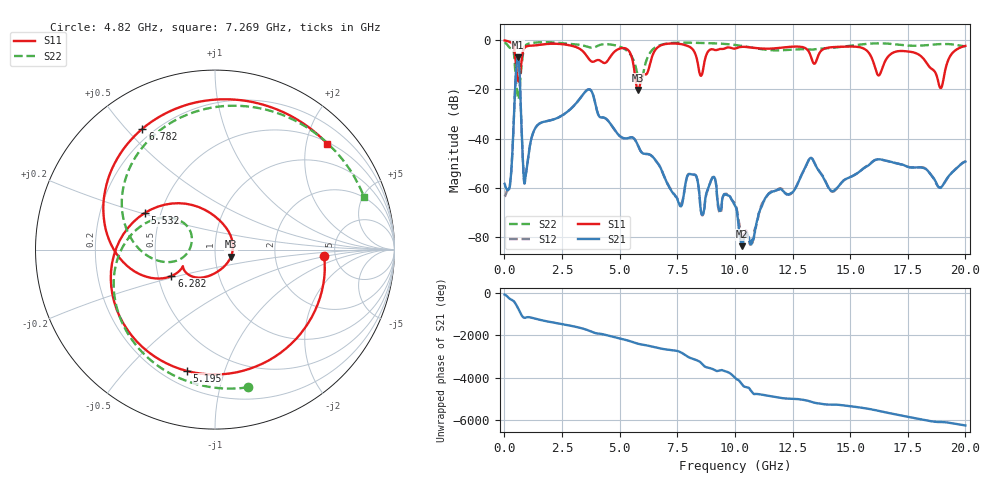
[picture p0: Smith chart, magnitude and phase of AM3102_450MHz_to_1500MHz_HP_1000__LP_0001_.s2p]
!Agilent Technologies,E8364B,MY43040894,A.07.50.67
!Agilent E8364B: A.07.50.67
!Date: Thursday, January 11, 2018 05:56:26
!Correction: S11(Full 2 Port(1,2))
!S21(Full 2 Port(1,2))
!S12(Full 2 Port(1,2))
!S22(Full 2 Port(1,2))
!S2P File: Measurements: S11, S21, S12, S22:
# Hz S  dB  R 50
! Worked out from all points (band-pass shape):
!   1601 points, 10 MHz to 20 GHz, reference 50 ohm
!   highest |S21| = -6.99 dB at 584.7 MHz (marker M1); lowest = -83.8 dB at 10.3 GHz (marker M2)
!   |S21| within 3 dB of the highest: 531.9 MHz to 640.9 MHz (109 MHz wide, 18.6 % of centre)
!   lowest |S11| = -20.2 dB at 5.807 GHz (marker M3), VSWR 1.22, Z = 59.5 - j4.79 ohm
!   |S11| at or under -10 dB: 5.6 GHz to 6.307 GHz (707.1 MHz wide, 11.9 % of centre); 16.05 GHz to 16.45 GHz (401 MHz wide, 2.47 % of centre); 18.37 GHz to 19.18 GHz (811.9 MHz wide, 4.32 % of centre)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
!   |S22| runs from -24.1 to -0.8 dB; largest |S21 - S12| = 0.002
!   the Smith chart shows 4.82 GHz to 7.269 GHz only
!   S11 on the Smith chart (normalised r, x): 4.82 GHz: 4.06, -0.48; 5.195 GHz: 0.29, -0.75; 5.532 GHz: 0.41, +0.21; 6.282 GHz: 0.59, -0.19; 6.782 GHz: 0.16, +0.56; 7.269 GHz: 0.53, +2.42
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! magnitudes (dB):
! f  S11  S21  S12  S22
! 10 MHz  -0.1  -58.4  -63.5  -0.8
! 259.9 MHz  -0.8  -57.5  -57.5  -3.2
! 584.7 MHz  -16.2  -7.0  -7.0  -23.3
! 909.5 MHz  -2.7  -56.0  -55.9  -2.1
! 1.397 GHz  -2.0  -35.0  -35.0  -0.9
! 3.346 GHz  -4.0  -22.9  -22.9  -2.0
! 4.82 GHz  -4.3  -37.0  -37.0  -2.1
! 5.195 GHz  -3.2  -39.9  -39.9  -3.4
! 5.532 GHz  -7.1  -39.5  -39.5  -6.7
! 5.807 GHz  -20.2  -43.1  -43.2  -15.5
! 6.282 GHz  -10.9  -46.4  -46.4  -5.6
! 6.682 GHz  -2.6  -50.4  -50.4  -2.2
! 6.782 GHz  -2.1  -52.0  -52.0  -1.9
! 7.269 GHz  -1.3  -61.7  -61.5  -1.1
! 8.531 GHz  -14.4  -69.7  -69.8  -1.1
! 10.01 GHz  -3.4  -67.3  -66.8  -1.9
! 10.3 GHz  -2.7  -83.8  -79.8  -2.3
! 13.34 GHz  -7.8  -48.1  -48.0  -3.8
! 14.24 GHz  -2.8  -61.4  -61.6  -3.1
! 16.68 GHz  -6.3  -49.3  -49.3  -1.4
! 18.93 GHz  -19.5  -60.1  -59.9  -1.5
! 20 GHz  -2.3  -49.4  -49.2  -2.5
